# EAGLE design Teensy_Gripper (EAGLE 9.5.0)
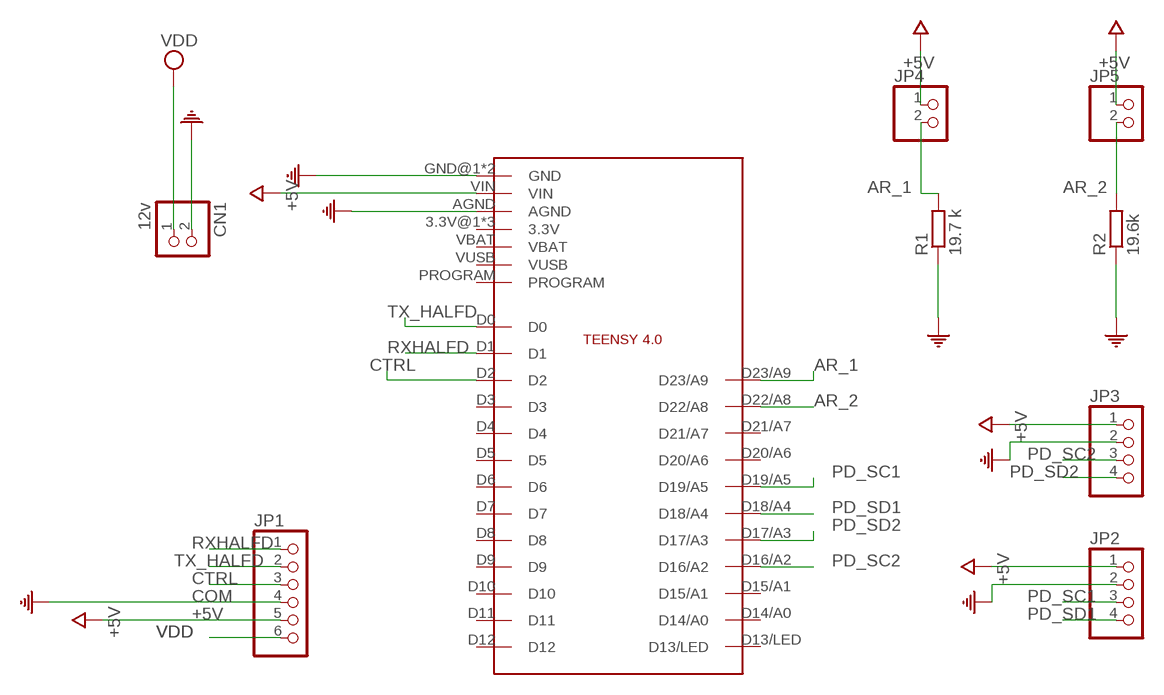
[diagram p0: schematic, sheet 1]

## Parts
CN1  12v  JST_2PIN-THM-RA  [JST-PH-2-THM-RA]
JP1  PINHD-1X6  [1X06]
JP2  PINHD-1X4  [1X04]
JP3  PINHD-1X4  [1X04]
JP4  PINHD-1X2  [1X02]
JP5  PINHD-1X2  [1X02]
R1  19.7 k  R-EU_0207/10  [0207/10]
R2  19.6k  R-EU_0207/10  [0207/10]
U$1  TEENSY4.0  [TEENSY4.0]

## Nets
+5V: JP1.5 JP2.1 JP3.1 JP4.1 JP5.1 U$1.VIN
AR_1: JP4.2 R1.2 U$1.D23/A9
AR_2: JP5.2 R2.2 U$1.D22/A8
COM: CN1.2 JP1.4 JP2.2 JP3.2 R1.1 R2.1 U$1.AGND U$1.GND@1(GND) U$1.GND@2(GND)
CTRL: JP1.3 U$1.D2
PD_SC1: JP2.3 U$1.D19/A5
PD_SC2: JP3.3 U$1.D16/A2
PD_SD1: JP2.4 U$1.D18/A4
PD_SD2: JP3.4 U$1.D17/A3
RXHALFD: JP1.1 U$1.D1
TX_HALFD: JP1.2 U$1.D0
VDD: CN1.1 JP1.6
Unconnected: U$1.3.3V@1(3.3V) U$1.3.3V@2(3.3V) U$1.D3 U$1.D4 U$1.D5 U$1.D6 U$1.D7 U$1.D8 U$1.D9 U$1.D10 U$1.D11 U$1.D12 U$1.D13/LED U$1.D14/A0 U$1.D15/A1 U$1.D20/A6 U$1.D21/A7 U$1.ON/OFF(3.3V) U$1.PROGRAM U$1.VBAT U$1.VUSB

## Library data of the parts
CN1 = adafruit:JST_2PIN: JST 2-Pin Connectors of various flavors
JP1 = pinhead:PINHD-1X6: PIN HEADER
JP2 JP3 = pinhead:PINHD-1X4: PIN HEADER
JP4 JP5 = pinhead:PINHD-1X2: PIN HEADER
R1 R2 = rcl:R-EU_: RESISTOR, European symbol; SPICEPREFIX: R
U$1 = Teensy4.0:TEENSY4.0

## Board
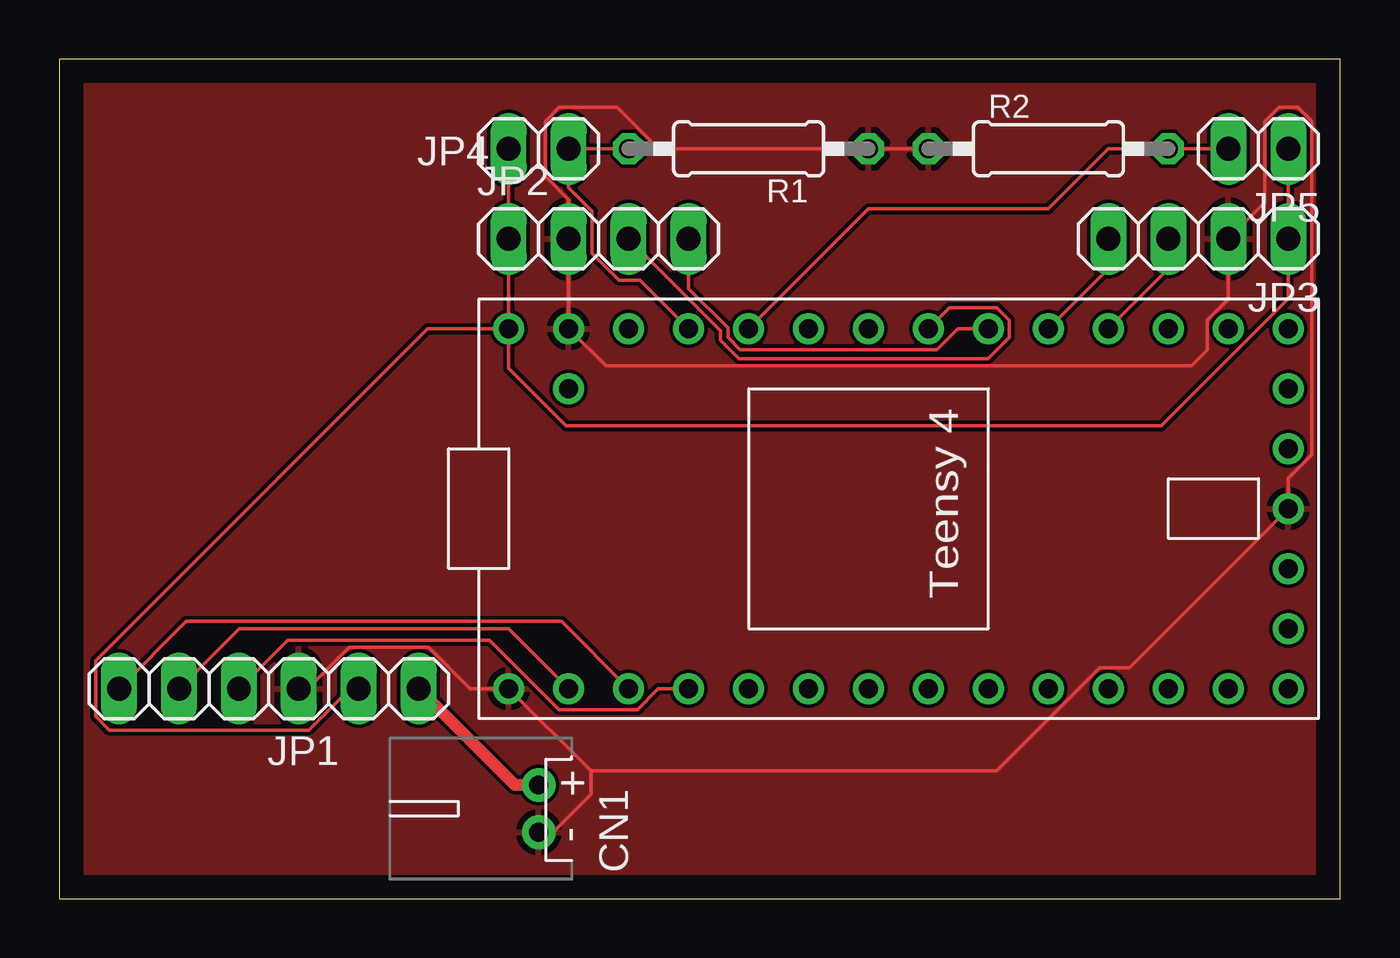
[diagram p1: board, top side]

Size 54.28 x 35.55 mm. Coordinates in mm from the lower left corner, seen from the top.
Outline: 0,0 54.28,0 54.28,35.55 0,35.55 0,0
Copper layers (1*16): Top 0.035mm / dielectric 1.5mm / Bottom 0.035mm
Design rules "default": minimum track width 6mil, minimum drill 0.35mm, track to track 6mil, track to pad 6mil, pad to pad 6mil, via to via 6mil, smd to smd 6mil, copper to edge 40mil, drill to drill 6mil, minimum pad ring 10mil, minimum via ring 8mil, stop-mask expansion 4mil, vias tented up to drill 0mil, thermal gap 10mil

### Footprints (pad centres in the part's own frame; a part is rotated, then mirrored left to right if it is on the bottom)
JST-PH-2-THM-RA = drill 0.8 pad 1.422: 1 1,0; 2 -1,0
1X06 = drill 1.016 long: 1 -6.35,0; 2 -3.81,0; 3 -1.27,0; 4 1.27,0; 5 3.81,0; 6 6.35,0
1X04 = drill 1.016 long: 1 -3.81,0; 2 -1.27,0; 3 1.27,0; 4 3.81,0
1X02 = drill 1.016 long: 1 -1.27,0; 2 1.27,0
0207/10 = drill 0.813 octagon: 1 -5.08,0; 2 5.08,0
TEENSY4.0 = drill 0.8: 3.3V@1 7.62,10.16; 3.3V@2 -2.54,-17.78; AGND 7.62,12.7; D0 -7.62,12.7; D1 -7.62,10.16; D2 -7.62,7.62; D3 -7.62,5.08; D4 -7.62,2.54; D5 -7.62,0; D6 -7.62,-2.54; D7 -7.62,-5.08; D8 -7.62,-7.62; D9 -7.62,-10.16; D10 -7.62,-12.7; D11 -7.62,-15.24; D12 -7.62,-17.78; D13/LED 7.62,-17.78; D14/A0 7.62,-15.24; D15/A1 7.62,-12.7; D16/A2 7.62,-10.16; D17/A3 7.62,-7.62; D18/A4 7.62,-5.08; D19/A5 7.62,-2.54; D20/A6 7.62,0; D21/A7 7.62,2.54; D22/A8 7.62,5.08; D23/A9 7.62,7.62; GND@1 -7.62,15.24; GND@2 0,-17.78; ON/OFF 5.08,-17.78; PROGRAM 2.54,-17.78; VBAT -5.08,-17.78; VIN 7.62,15.24; VUSB 5.08,12.7

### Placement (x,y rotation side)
CN1  20.32,3.81 90 top
JP1  8.89,8.89 0 top
JP2  22.86,27.94 0 top
JP3  48.26,27.94 180 top
JP4  20.32,31.75 0 top
JP5  50.8,31.75 180 top
R1  29.21,31.75 180 top
R2  41.91,31.75 0 top
U$1  34.29,16.51 90 top

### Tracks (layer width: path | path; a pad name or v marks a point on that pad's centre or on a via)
+5V
  Top 0.152: U$1.VIN JP2.1 JP4.1 | 51.69,31.75 JP5.1 JP3.1 52.07,25.4 46.69,20.02 21.49,20.02 19.05,22.45 U$1.VIN | JP1.5 12.32,8.89 10.57,7.14 2.13,7.14 1.55,7.72 1.55,10.06 15.62,24.13 U$1.VIN
AR_1
  Top 0.152: R1.2 JP4.2 21.59,30.1 22.58,29.11 22.58,27.33 23.72,26.19 24.61,26.19 U$1.D23/A9
AR_2
  Top 0.152: JP5.2 R2.2 44.45,31.75 41.91,29.21 34.29,29.21 U$1.D22/A8
COM
  Top 0.152: R2.1 R1.1 25.39,31.75 23.64,33.5 21.18,33.5 20.6,32.92 20.6,30.58 21.59,29.59 JP2.2 U$1.AGND 23.16,22.55 47.95,22.55 48.65,23.25 48.65,24.5 49.53,25.38 JP3.2 51.08,29.49 51.08,32.92 51.66,33.5 52.48,33.5 53.06,32.92 53.06,18.79 52.07,17.8 U$1.GND@2 45.33,9.77 44.08,9.77 39.72,5.41 22.53,5.41 | JP1.4 10.54,8.89 12.29,10.64 15.65,10.64 17.4,8.89 U$1.GND@1 22.53,5.41 | CN1.2 20.92,2.81 22.53,4.42 22.53,5.41
  pour Top: 0,35.56 0,0 54.61,0 54.61,35.56
CTRL
  Top 0.152: JP1.3 9.68,10.95 18.24,10.95 21.18,8.01 24.5,8.01 25.38,8.89 U$1.D2
PD_SC1
  Top 0.152: 36.81,24.13 U$1.D19/A5 37.71,25.01 39.74,25.01 40.25,24.5 40.25,23.76 39.35,22.86 28.8,22.86 28.02,23.64 28.02,24.05 JP2.3
PD_SC2
  Top 0.152: JP3.3 46.99,26.67 U$1.D16/A2
PD_SD1
  Top 0.152: 39.35,24.13 U$1.D18/A4 38.08,24.13 37.2,23.25 28.84,23.25 28.33,23.76 28.33,24.17 26.67,25.83 JP2.4
PD_SD2
  Top 0.152: JP3.4 44.45,26.67 U$1.D17/A3
RXHALFD
  Top 0.152: JP1.1 5.38,11.73 21.29,11.73 U$1.D1
TX_HALFD
  Top 0.152: JP1.2 7.62,11.43 19.05,11.43 U$1.D0
VDD
  Top 0.508: CN1.1 19.32,4.81 JP1.6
